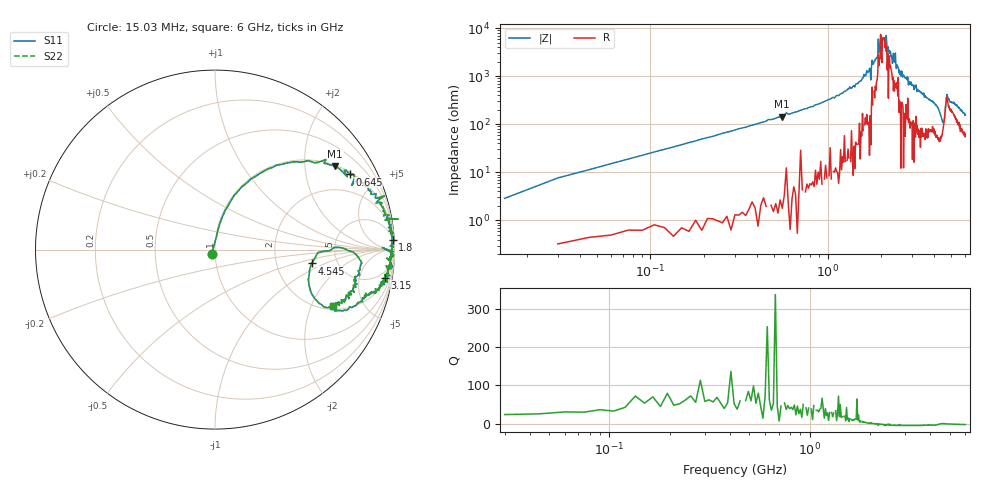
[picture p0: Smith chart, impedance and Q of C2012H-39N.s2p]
!	Network	Analyzer	HP8753E.07.74:	Oct	30	2002	Serial	No.	JP38451487
!	Hewlett-Packard
!	28	Aug	2009	10:12:14
!	Frequency	S11	S21	S12	S22
#	HZ	S	RI	R	50
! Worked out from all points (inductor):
!   400 points, 15.03 MHz to 6 GHz, reference 50 ohm
!   read as one part in series: L = 40.1 nH near 45.03 MHz
!   highest Q = 70.9 at 555 MHz (marker M1), where L = 41 nH
!   self-resonance near 2.085 GHz
!   S11 on the Smith chart (normalised r, x): 15.03 MHz: 0.96, -0.04; 645 MHz: 1.10, +3.52; 1.8 GHz: 6, +35; 3.15 GHz: 3, -11; 4.545 GHz: 3.22, -0.71; 6 GHz: 2.14, -2.90
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1.502992e7  -0.0177 -0.0224  1.02 0.0224  1.02 0.0224  -0.0177 -0.0224
6.00297e7  0.0273 0.147  0.973 -0.147  0.973 -0.147  0.0273 0.147
1.500292e8  0.129 0.326  0.871 -0.326  0.871 -0.326  0.129 0.326
5.550272e8  0.67 0.464  0.33 -0.464  0.33 -0.464  0.67 0.464
6.450268e8  0.75 0.419  0.25 -0.419  0.25 -0.419  0.75 0.419
1.020025e9  0.909 0.275  0.0911 -0.275  0.0911 -0.275  0.909 0.275
1.725021e9  0.994 0.068  0.00571 -0.068  0.00571 -0.068  0.994 0.068
1.755021e9  0.981 0.117  0.0193 -0.117  0.0193 -0.117  0.981 0.117
1.800021e9  0.989 0.0548  0.0111 -0.0548  0.0111 -0.0548  0.989 0.0548
1.90502e9  0.984 0.0381  0.0161 -0.0381  0.0161 -0.0381  0.984 0.0381
1.93502e9  0.992 0.0146  0.00827 -0.0146  0.00827 -0.0146  0.992 0.0146
2.01002e9  0.987 0.0162  0.013 -0.0162  0.013 -0.0162  0.987 0.0162
2.145019e9  0.993 -0.0124  0.00668 0.0124  0.00668 0.0124  0.993 -0.0124
2.175019e9  0.933 0.0117  0.0673 -0.0117  0.0673 -0.0117  0.933 0.0117
2.190019e9  0.983 -0.0164  0.0171 0.0164  0.0171 0.0164  0.983 -0.0164
3.015015e9  0.974 -0.145  0.0257 0.145  0.0257 0.145  0.974 -0.145
3.150014e9  0.948 -0.158  0.052 0.158  0.052 0.158  0.948 -0.158
4.00501e9  0.832 -0.273  0.168 0.273  0.168 0.273  0.832 -0.273
4.545007e9  0.539 -0.0773  0.461 0.0773  0.461 0.0773  0.539 -0.0773
4.725006e9  0.818 -0.0736  0.182 0.0736  0.182 0.0736  0.818 -0.0736
5.010005e9  0.783 -0.166  0.217 0.166  0.217 0.166  0.783 -0.166
6e9  0.656 -0.317  0.344 0.317  0.344 0.317  0.656 -0.317
